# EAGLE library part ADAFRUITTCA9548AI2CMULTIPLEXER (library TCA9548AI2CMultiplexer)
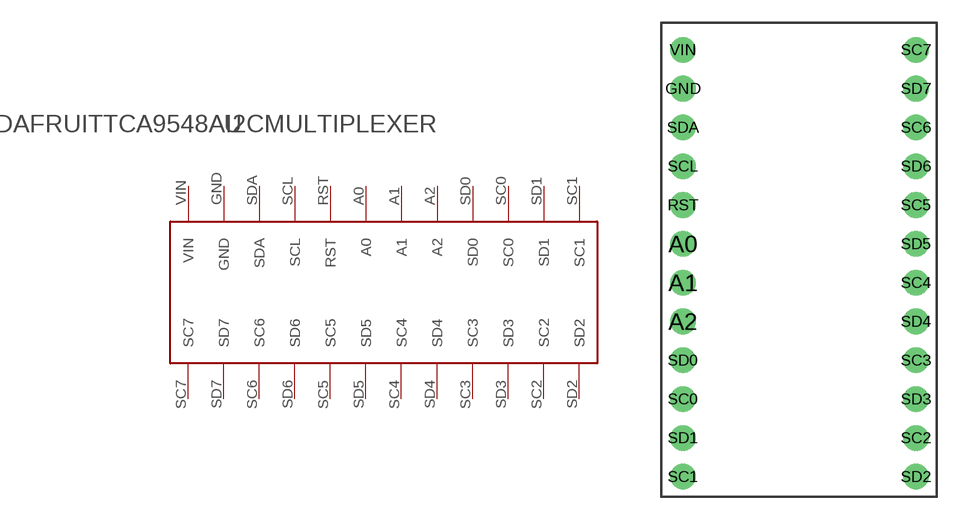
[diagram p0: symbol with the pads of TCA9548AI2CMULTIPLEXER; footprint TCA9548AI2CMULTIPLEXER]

Designator prefix -

## ADAFRUITTCA9548AI2CMULTIPLEXER  [TCA9548AI2CMULTIPLEXER]
A0  A0
A1  A1
A2  A2
GND  GND
RST  RST
SC0  SC0
SC1  SC1
SC2  SC2
SC3  SC3
SC4  SC4
SC5  SC5
SC6  SC6
SC7  SC7
SCL  SCL
SD0  SD0
SD1  SD1
SD2  SD2
SD3  SD3
SD4  SD4
SD5  SD5
SD6  SD6
SD7  SD7
SDA  SDA
VIN  VIN

## Footprint TCA9548AI2CMULTIPLEXER (pad centres in mm)
drill 1 pad 1.676: A0 -8.59,2.54; A1 -8.59,0; A2 -8.59,-2.54; GND -8.59,12.7; RST -8.59,5.08; SC0 -8.59,-7.62; SC1 -8.59,-12.7; SC2 6.65,-10.16; SC3 6.65,-5.08; SC4 6.65,0; SC5 6.65,5.08; SC6 6.65,10.16; SC7 6.65,15.24; SCL -8.59,7.62; SD0 -8.59,-5.08; SD1 -8.59,-10.16; SD2 6.65,-12.7; SD3 6.65,-7.62; SD4 6.65,-2.54; SD5 6.65,2.54; SD6 6.65,7.62; SD7 6.65,12.7; SDA -8.59,10.16; VIN -8.59,15.24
